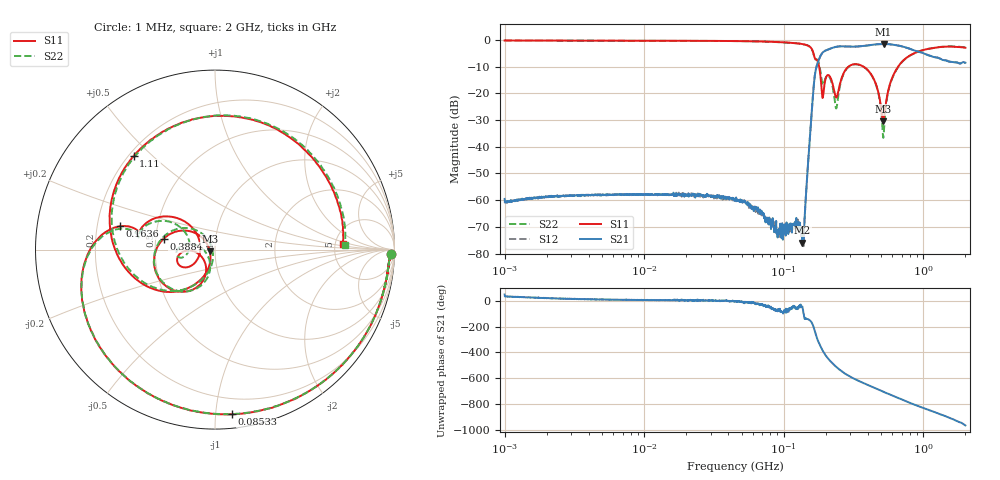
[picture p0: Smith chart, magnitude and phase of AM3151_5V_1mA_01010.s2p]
! Date/Time: Fri Jun 26 10:47:31 2020
! Network Analyzer:  Rev:
! Sweep from 1000000.0 to 2000000000.0, 1601 Points ! Power Supply: 0 V, 0 A
# HZ S DB R 50
!freq MagS11 AngS11 MagS21 AngS21 MagS12 AngS12 MagS22 AngS22
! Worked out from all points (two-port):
!   1601 points, 1 MHz to 2 GHz, reference 50 ohm
!   highest |S21| = -1.49 dB at 518.9 MHz (marker M1); lowest = -75.9 dB at 135.9 MHz (marker M2)
!   |S21| within 3 dB of the highest: 191.8 MHz to 940.2 MHz (748.5 MHz wide, 132 % of centre)
!   lowest |S11| = -30.4 dB at 516.5 MHz (marker M3), VSWR 1.06, Z = 47.2 - j0.837 ohm
!   |S11| at or under -10 dB: 179.2 MHz to 290.3 MHz (111.1 MHz wide, 47.3 % of centre); 372.8 MHz to 659.1 MHz (286.3 MHz wide, 55.5 % of centre)
!   |S22| runs from -36.7 to -0.2 dB; largest |S21 - S12| = 0.0088
!   S11 on the Smith chart (normalised r, x): 1 MHz: 36, -48; 85.33 MHz: 0.09, -1.10; 163.6 MHz: 0.30, +0.11; 388.4 MHz: 0.55, +0.07; 1.11 GHz: 0.22, +0.44; 2 GHz: 5.91, +0.75
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1000000  -0.17 -1.5  -59.53 47.6  -60.59 31.5  -0.17 -1.5
3555161  -0.25 -3.9  -58.05 12.8  -58.12 11.3  -0.24 -3.9
1.263916e7  -0.28 -12.7  -57.78 4.7  -58.06 4.4  -0.28 -12.7
4.493426e7  -0.40 -44.6  -60.21 -1.8  -60.30 -5.5  -0.41 -44.5
8.533003e7  -0.71 -84.3  -71.99 -71.6  -69.21 -67.9  -0.72 -84.3
1.35922e8  -1.52 -140.4  -75.89 -44.8  -72.76 -32.3  -1.53 -140.3
1.589914e8  -3.43 176.8  -26.07 -171.8  -26.06 -171.9  -3.48 177.3
1.635886e8  -5.24 166.3  -17.68 155.8  -17.68 155.7  -5.40 167.5
1.756708e8  -8.21 154.4  -8.32 51.1  -8.31 51.1  -7.79 160.9
1.877516e8  -20.06 150.5  -5.03 -15.2  -5.00 -15.2  -15.71 156.1
2.144628e8  -13.77 -171.1  -3.28 -104.4  -3.27 -104.4  -14.23 174.8
2.369614e8  -21.51 -149.4  -2.55 -150.5  -2.56 -150.6  -25.64 -153.5
2.618205e8  -13.75 -112.6  -2.36 171.6  -2.35 171.6  -14.05 -108.9
3.883688e8  -10.67 168.1  -2.12 74.5  -2.13 74.6  -10.74 164.8
4.586222e8  -16.76 140.3  -1.65 40.8  -1.64 40.9  -16.88 133.2
5.164555e8  -30.42 -162.9  -1.50 16.5  -1.50 16.3  -36.65 -165.5
5.189154e8  -30.13 -152.4  -1.49 15.5  -1.50 15.5  -35.74 -144.3
5.652395e8  -18.10 -109.9  -1.57 -2.2  -1.57 -2.2  -18.44 -105.5
7.69728e8  -6.38 -161.7  -2.99 -62.8  -3.00 -62.8  -6.46 -163.6
1.109683e9  -3.21 131.0  -5.87 -126.9  -5.87 -126.9  -3.21 127.6
1.482693e9  -2.46 73.4  -7.85 -178.7  -7.73 -179.0  -2.40 70.5
2e9  -2.92 2.5  -8.52 115.5  -8.69 115.0  -2.80 2.1
